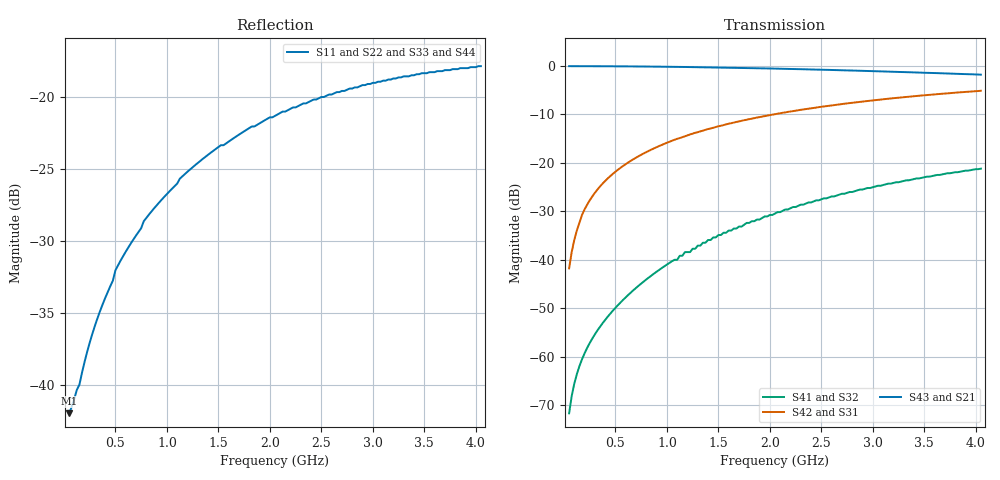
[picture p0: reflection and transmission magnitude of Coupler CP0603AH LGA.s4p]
!	AVX THIN FILM OPERATION
!	CP0603 HIGH DIRECTIVITY COUPLERS
!	P/N CP0603AxxxxHLTR
!	Network	Analyzer HP8720ES.07.64:Feb23,2000 Serial No.US39172382
!	Hewlett-Packard
!	24 July 2003	02:45:57
# MHZ S MA R 50
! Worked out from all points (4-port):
!   161 points, 50 MHz to 4.05 GHz, reference 50 ohm
!   strongest paths, dB at 50 MHz, 1.05 GHz, 2.05 GHz, 3.05 GHz, 4.05 GHz:
!     S43: -0.1, -0.2, -0.6, -1.1, -1.8
!     S21: -0.1, -0.2, -0.6, -1.1, -1.8
!     S42: -41.8, -15.4, -10.0, -7.0, -5.1
!     S31: -41.8, -15.4, -10.0, -7.0, -5.1
!     S41: -71.7, -40.3, -30.5, -24.7, -21.2
!     S32: -71.7, -40.3, -30.5, -24.7, -21.2
!   lowest |S11| = -42.0 dB at 50 MHz (marker M1), VSWR 1.02, Z = 50.8 - j0.244 ohm
!   |S11| at or under -10 dB: start of sweep to end of sweep
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50  0.007952 -17.6  0.992 -0.3  0.008151 89.6  0.0002611 85.1
    0.992 -0.3  0.007952 -17.6  0.0002611 85.1  0.008151 89.6
    0.008151 89.6  0.0002611 85.1  0.007952 -17.6  0.992 -0.3
    0.0002611 85.1  0.008151 89.6  0.992 -0.3  0.007952 -17.6
100  0.008929 -32.5  0.992 -0.7  0.016 89.3  0.0005264 80.6
     0.992 -0.7  0.008929 -32.5  0.0005264 80.6  0.016 89.3
     0.016 89.3  0.0005264 80.6  0.008929 -32.5  0.992 -0.7
     0.0005264 80.6  0.016 89.3  0.992 -0.7  0.008929 -32.5
175  0.011 -48.6  0.992 -1.2  0.029 88.8  0.0009403 73.9
     0.992 -1.2  0.011 -48.6  0.0009403 73.9  0.029 88.8
     0.029 88.8  0.0009403 73.9  0.011 -48.6  0.992 -1.2
     0.0009403 73.9  0.029 88.8  0.992 -1.2  0.011 -48.6
350  0.018 -67.9  0.991 -2.4  0.057 87.5  0.002039 59.7
     0.991 -2.4  0.018 -67.9  0.002039 59.7  0.057 87.5
     0.057 87.5  0.002039 59.7  0.018 -67.9  0.991 -2.4
     0.002039 59.7  0.057 87.5  0.991 -2.4  0.018 -67.9
1175  0.054 -91.1  0.973 -8.1  0.188 81.8  0.012 19.7
      0.973 -8.1  0.054 -91.1  0.012 19.7  0.188 81.8
      0.188 81.8  0.012 19.7  0.054 -91.1  0.973 -8.1
      0.012 19.7  0.188 81.8  0.973 -8.1  0.054 -91.1
2375  0.096 -103.1  0.919 -15.8  0.362 74.0  0.039 -4.7
      0.919 -15.8  0.096 -103.1  0.039 -4.7  0.362 74.0
      0.362 74.0  0.039 -4.7  0.096 -103.1  0.919 -15.8
      0.039 -4.7  0.362 74.0  0.919 -15.8  0.096 -103.1
4050  0.128 -113.2  0.811 -25.4  0.553 64.6  0.087 -23.0
      0.811 -25.4  0.128 -113.2  0.087 -23.0  0.553 64.6
      0.553 64.6  0.087 -23.0  0.128 -113.2  0.811 -25.4
      0.087 -23.0  0.553 64.6  0.811 -25.4  0.128 -113.2
